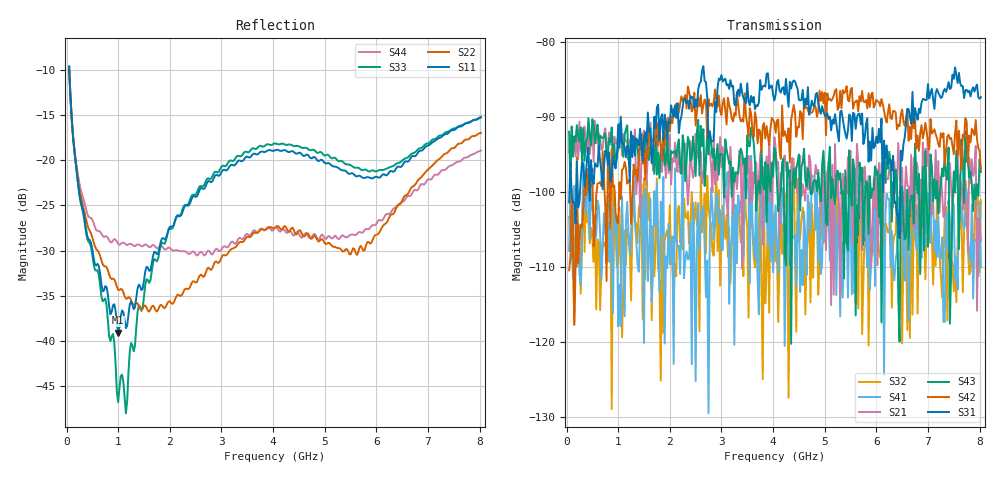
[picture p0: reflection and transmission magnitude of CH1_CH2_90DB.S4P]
!Agilent Technologies,E5071C,MY46316741,A.11.02
!Date: Thu May 28 14:55:32 2026
!Data & Calibration Information:
!1:CH1 INPUT 2:CH1 OUTPUT 3:CH2 INPUT 4:CH2 OUTPUT
!Freq	S11:SOLT4(ON)	S12:SOLT4(ON)	S13:SOLT4(ON)	S14:SOLT4(ON)
!	S21:SOLT4(ON)	S22:SOLT4(ON)	S23:SOLT4(ON)	S24:SOLT4(ON)
!	S31:SOLT4(ON)	S32:SOLT4(ON)	S33:SOLT4(ON)	S34:SOLT4(ON)
!	S41:SOLT4(ON)	S42:SOLT4(ON)	S43:SOLT4(ON)	S44:SOLT4(ON)
!PortZ  Port1:50+j0  Port2:50+j0  Port3:50+j0  Port4:50+j0
!Above PortZ is port z conversion or system Z0 setting when saving the data.
!When reading, reference impedance value at option line is always used.
# Hz S dB R 50
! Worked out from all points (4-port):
!   320 points, 50 MHz to 8.025 GHz, reference 50 ohm
!   strongest paths, dB at 50 MHz, 2.05 GHz, 4.05 GHz, 6.05 GHz, 8.025 GHz:
!     S31: -101.4, -89.4, -87.0, -91.6, -87.4
!     S42: -110.4, -90.8, -92.1, -88.0, -96.9
!     S43: -92.0, -94.8, -94.8, -103.3, -97.3
!     S21: -94.7, -95.5, -94.1, -96.1, -106.5
!     S41: -107.8, -105.9, -101.8, -102.5, -110.0
!     S32: -103.3, -109.4, -109.2, -107.8, -101.1
!   lowest |S11| = -39.1 dB at 1 GHz (marker M1), VSWR 1.02, Z = 49.1 - j0.632 ohm
!   |S11| at or under -10 dB: 52.92 MHz to end of sweep
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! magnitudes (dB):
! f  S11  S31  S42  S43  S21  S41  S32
! 50 MHz  -9.6  -101.4  -110.4  -92.0  -94.7  -107.8  -103.3
! 400 MHz  -28.3  -95.4  -96.9  -92.8  -94.7  -98.7  -104.0
! 1 GHz  -39.1  -91.0  -104.2  -94.4  -92.5  -117.9  -109.4
! 1.7 GHz  -30.1  -90.0  -93.8  -97.6  -95.1  -99.9  -111.2
! 3.025 GHz  -21.1  -85.3  -88.2  -95.1  -94.0  -107.7  -101.9
! 5.625 GHz  -21.8  -90.1  -87.8  -101.7  -93.6  -96.0  -100.9
! 8.025 GHz  -15.2  -87.4  -96.9  -97.3  -106.5  -110.0  -101.1
